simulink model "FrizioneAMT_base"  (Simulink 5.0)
settings: Solver=ode45  StartTime=0.0  StopTime=10.0  RelTol=1e-6  AbsTol=1e-6
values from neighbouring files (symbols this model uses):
  Af = 2*10^(-4)*m^2    (= 0.0002)    [FrizioneAMT.m]
  bv = 80*N*secondi/m    (= 80)    [FrizioneAMT.m]
  dv = 0.5    [FrizioneAMT.m]
  Istep = 0.5*Amp    (= 0.5)    [FrizioneAMT.m]
  Ke = Fnom/corsanom    (= 50000)    [FrizioneAMT.m]
  Ki = 50*bar/Amp    (= 5000000)    [FrizioneAMT.m]
  Kq = 1.5*bar/lmin    (= 9000000000)    [FrizioneAMT.m]
  m1 = 2*Kg    (= 2)    [FrizioneAMT.m]
  tauv = 16*msec    (= 0.016)    [FrizioneAMT.m]
  Wnv = 1200*rad/secondi    (= 1200)    [FrizioneAMT.m]
  x0 = 0*m    (= 0)    [FrizioneAMT.m]
  xp0 = 0.2*m/secondo    (= 0.2)    [FrizioneAMT.m]

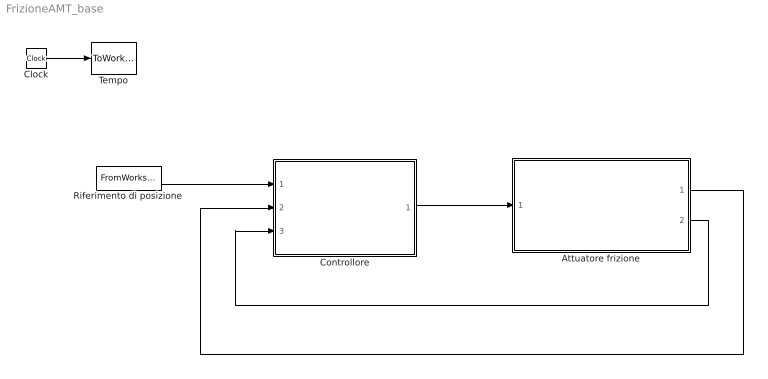
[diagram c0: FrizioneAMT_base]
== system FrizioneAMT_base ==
  Attuatore frizione : Subsystem
  Clock : Clock
  Controllore : Subsystem
  Riferimento di posizione : FromWorkspace  VariableName=[tsim xr]  SampleTime=0
  Tempo : ToWorkspace  VariableName=t  SampleTime=-1  SaveFormat=Array
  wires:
  Clock/1 -> Tempo/1
  Controllore/1(corrente) -> Attuatore frizione/1(Corrente di  controllo)
  Riferimento di posizione/1 -> Controllore/1(Riferimento)
  Attuatore frizione/2(Pressione) -> Controllore/3(Pressione)
  Attuatore frizione/1(Posizione) -> Controllore/2(Posizione)

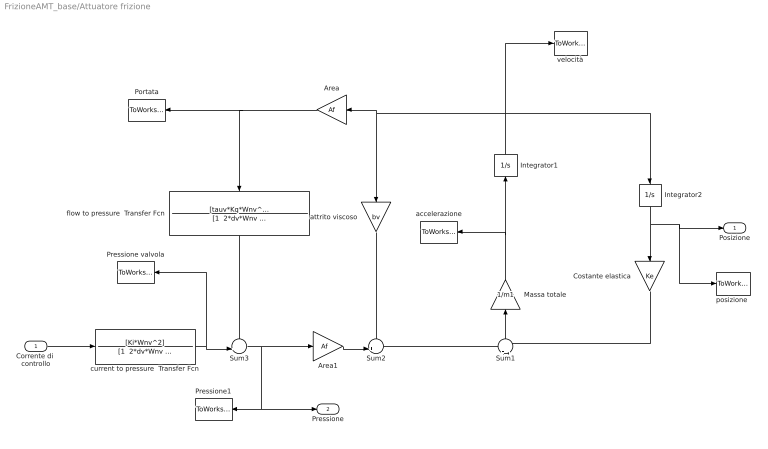
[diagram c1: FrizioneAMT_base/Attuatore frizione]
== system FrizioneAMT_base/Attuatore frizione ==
  Corrente di  controllo : Inport
  Area : Gain  Orientation=left  Gain=Af
  Area1 : Gain  Gain=Af
  Costante elastica : Gain  Orientation=down  Gain=Ke
  Integrator1 : Integrator  Orientation=up  InitialCondition=xp0
  Integrator2 : Integrator  Orientation=down  InitialCondition=x0
  Massa totale : Gain  Orientation=up  Gain=1/m1
  Portata : ToWorkspace  VariableName=Qx  SampleTime=-1  SaveFormat=Array
  Pressione valvola : ToWorkspace  VariableName=Pv  SampleTime=-1  SaveFormat=Array
  Pressione1 : ToWorkspace  VariableName=Px  SampleTime=-1  SaveFormat=Array
  Sum1 : Sum  Orientation=up  Inputs=+|-
  Sum2 : Sum  Inputs=-+|
  Sum3 : Sum  Inputs=-+|
  accelerazione : ToWorkspace  VariableName=xpp  SampleTime=-1  SaveFormat=Array
  attrito viscoso : Gain  Orientation=down  Gain=bv
  current to pressure  Transfer Fcn : TransferFcn  Numerator=[Ki*Wnv^2]  Denominator="[1  2*dv*Wnv  Wnv^2]"
  flow to pressure  Transfer Fcn : TransferFcn  Orientation=down  Numerator="[tauv*Kq*Wnv^2   Kq*Wnv^2]"  Denominator="[1  2*dv*Wnv  Wnv^2]"
  "posizione " : ToWorkspace  VariableName=x  SampleTime=-1  SaveFormat=Array
  velocità : ToWorkspace  VariableName=xp  SampleTime=-1  SaveFormat=Array
  Posizione : Outport
  Pressione : Outport  Port=2
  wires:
  Integrator1/1 -> velocità/1, attrito viscoso/1, Area/1, Integrator2/1
  attrito viscoso/1 -> Sum2/1
  Sum2/1 -> Sum1/1
  Sum1/1 -> Massa totale/1
  Costante elastica/1 -> Sum1/2
  Integrator2/1 -> Costante elastica/1, Posizione/1, "posizione "/1
  Area1/1 -> Sum2/2
  Sum3/1 -> Area1/1, Pressione/1, Pressione1/1
  Area/1 -> Portata/1, flow to pressure  Transfer Fcn/1
  current to pressure  Transfer Fcn/1 -> Sum3/2, Pressione valvola/1
  flow to pressure  Transfer Fcn/1 -> Sum3/1
  Corrente di  controllo/1 -> current to pressure  Transfer Fcn/1
  Massa totale/1 -> Integrator1/1, accelerazione/1

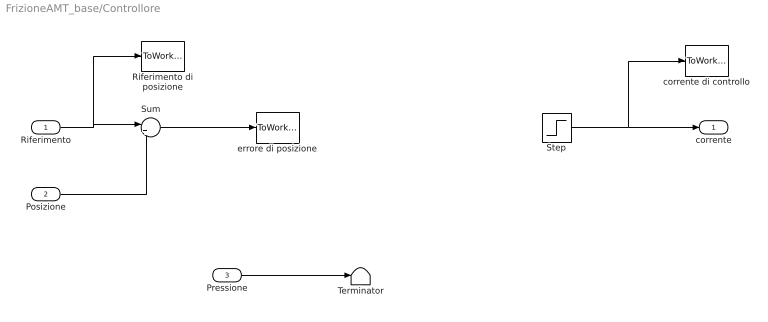
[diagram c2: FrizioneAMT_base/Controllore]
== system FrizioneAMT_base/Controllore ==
  Riferimento : Inport
  Posizione : Inport  Port=2
  Pressione : Inport  Port=3
  Riferimento di posizione : ToWorkspace  VariableName=xrif  SampleTime=-1  SaveFormat=Array
  Step : Step  Time=0.1  After=Istep  SampleTime=0
  Sum : Sum  Inputs=|+-
  Terminator : Terminator
  corrente di controllo : ToWorkspace  VariableName=Ic  SampleTime=-1  SaveFormat=Array
  errore di posizione : ToWorkspace  VariableName=ep  SampleTime=-1  SaveFormat=Array
  corrente : Outport
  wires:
  Step/1 -> corrente/1, corrente di controllo/1
  Riferimento/1 -> Sum/1, Riferimento di posizione/1
  Posizione/1 -> Sum/2
  Sum/1 -> errore di posizione/1
  Pressione/1 -> Terminator/1
